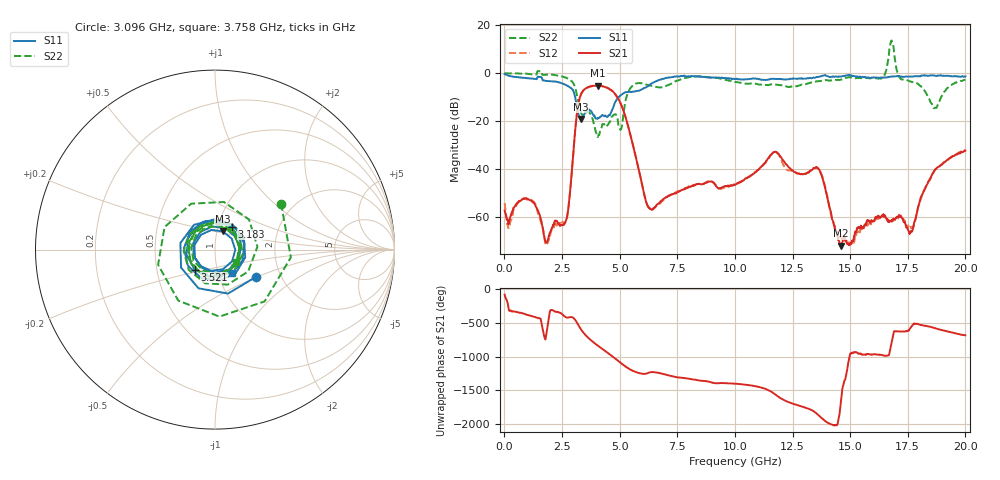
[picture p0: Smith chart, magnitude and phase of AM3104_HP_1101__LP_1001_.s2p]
!Created with skrf (http://scikit-rf.org).
# Hz S RI R 50.0
!freq ReS11 ImS11 ReS21 ImS21 ReS12 ImS12 ReS22 ImS22
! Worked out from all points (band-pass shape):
!   1601 points, 10 MHz to 20 GHz, reference 50 ohm
!   highest |S21| = -5.20 dB at 4.07 GHz (marker M1); lowest = -72.0 dB at 14.59 GHz (marker M2)
!   |S21| within 3 dB of the highest: 3.356 GHz to 4.755 GHz (1.398 GHz wide, 34.5 % of centre)
!   lowest |S11| = -19.1 dB at 3.308 GHz (marker M3), VSWR 1.25, Z = 53.4 + j11 ohm
!   |S11| at or under -10 dB: 3.07 GHz to 4.955 GHz (1.885 GHz wide, 47 % of centre)
!   |S22| runs from -26.7 to 13.6 dB; largest |S21 - S12| = 0.045
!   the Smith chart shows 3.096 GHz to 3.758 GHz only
!   S11 on the Smith chart (normalised r, x): 3.096 GHz: 1.50, -0.49; 3.183 GHz: 1.16, +0.30; 3.521 GHz: 0.78, -0.18; 3.758 GHz: 1.17, -0.31
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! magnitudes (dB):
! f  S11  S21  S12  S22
! 10 MHz  -0.4  -57.3  -54.2  -0.1
! 1.234 GHz  -2.3  -53.9  -53.5  -0.5
! 1.834 GHz  -3.3  -70.5  -71.4  -0.7
! 2.584 GHz  -4.6  -63.1  -62.7  -1.7
! 3.096 GHz  -11.2  -21.4  -21.4  -7.0
! 3.183 GHz  -16.0  -14.5  -14.5  -10.8
! 3.308 GHz  -19.1  -9.2  -9.3  -16.1
! 3.346 GHz  -18.8  -8.4  -8.5  -17.0
! 3.521 GHz  -16.0  -6.4  -6.5  -16.5
! 3.758 GHz  -15.8  -5.5  -5.5  -17.4
! 4.07 GHz  -18.7  -5.2  -5.3  -26.1
! 4.995 GHz  -9.6  -11.7  -11.7  -23.0
! 6.169 GHz  -5.8  -54.3  -54.3  -4.8
! 6.682 GHz  -3.0  -54.5  -54.9  -5.9
! 10.01 GHz  -2.5  -46.7  -46.5  -3.7
! 11.72 GHz  -2.4  -32.9  -33.0  -4.7
! 13.34 GHz  -2.1  -40.4  -40.3  -3.9
! 14.59 GHz  -1.4  -72.0  -68.3  -2.7
! 16.68 GHz  -1.6  -61.9  -61.6  7.2
! 17.65 GHz  -1.4  -65.8  -64.6  -3.6
! 18.66 GHz  -1.0  -40.5  -40.6  -14.5
! 20 GHz  -1.4  -32.4  -32.0  -2.8
